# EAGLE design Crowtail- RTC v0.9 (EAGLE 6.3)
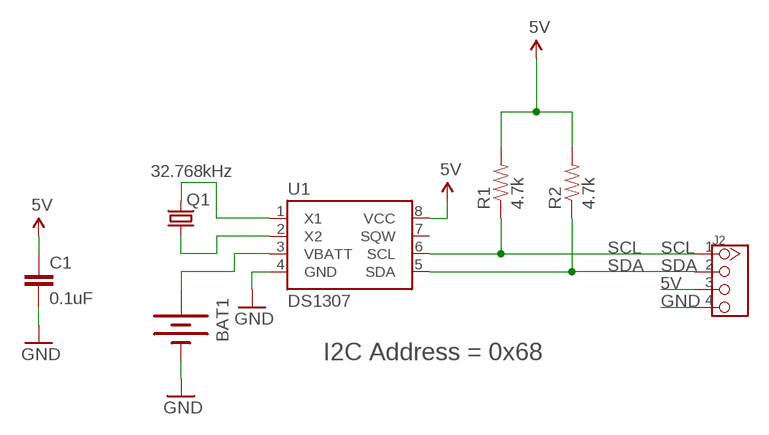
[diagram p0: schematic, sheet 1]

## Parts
BAT1  BATTERY12PTH  [BATTCON_12MM_PTH]
C1  0.1uF  0.1UF-25V(+80/-20%)(0603)  [0603-CAP]
J2  TWIG-4P-2.0-2.0  [4P-2.0]
Q1  32.768kHz  CRYSTAL32-SMD  [CRYSTAL-32KHZ-SMD]
R1  4.7k  4.7KOHM1/10W1%(0603)  [0603]
R2  4.7k  4.7KOHM1/10W1%(0603)  [0603]
U1  DS1307  DS1307SO8-TIGHT  [SO08-TIGHT]

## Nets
5V: C1.1 J2.3 R1.2 R2.2 U1.8(VCC)
GND: BAT1.GND(-) C1.2 J2.4 U1.4(GND)
N$1: Q1.X2 U1.1(X1)
N$2: Q1.X1 U1.2(X2)
N$4: BAT1.VCC@1(+) U1.3(VBATT)
SCL: J2.1 R1.1 U1.6(SCL)
SDA: J2.2 R2.1 U1.5(SDA)
Unconnected: U1.7(SQW)

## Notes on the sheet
- I2C Address = 0x68

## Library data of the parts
BAT1 = SparkFun-Electromechanical:BATTERY: Battery Holders
C1 = SparkFun-Capacitors:0.1UF-25V(+80/-20%)(0603): CAP-00810; PROD_ID: CAP-00810
J2 = Connector:TWIG-4P-2.0
Q1 = SparkFun-FreqCtrl:CRYSTAL: Various standard crystals. Proven footprints. Spark Fun Electronics SKU : COM-00534
R1 R2 = SparkFun-Resistors:4.7KOHM1/10W1%(0603): RES-07857; PROD_ID: RES-07857
U1 = SparkFun-FreqCtrl:DS1307: I2C real-time clock with battery backup.

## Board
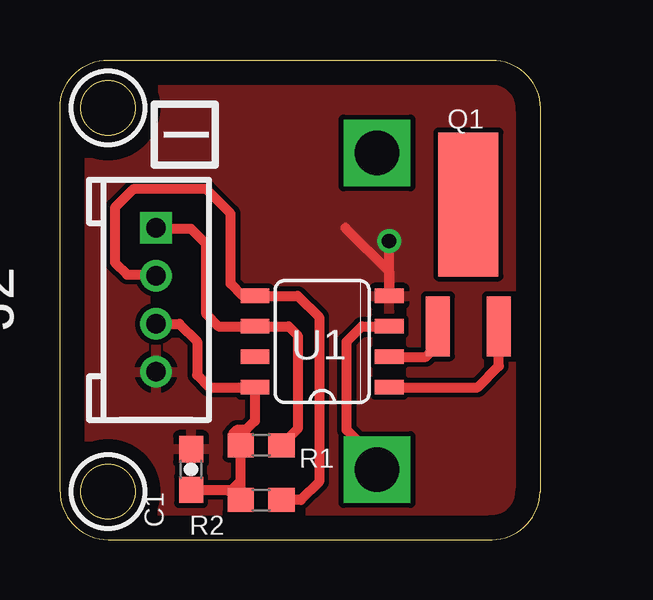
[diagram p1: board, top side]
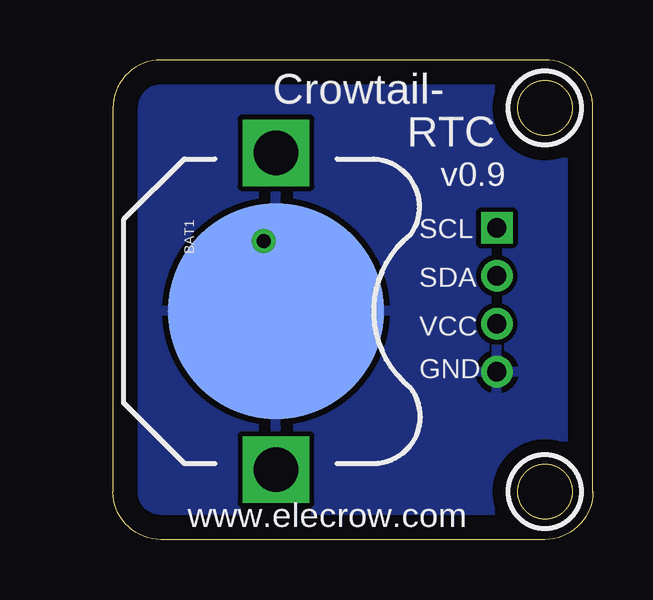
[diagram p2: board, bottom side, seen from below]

Size 20 x 20 mm. Coordinates in mm from the lower left corner, seen from the top.
Outline: 0,2 0,18 arc-90 2,20 18,20 arc-90 20,18 20,2 arc-90 18,0 2,0 arc-90 0,2
Outline: circle at 2,18 radius 1.14
Outline: circle at 2,2 radius 1.14
Copper layers (1*16): Top 0.035mm / dielectric 1.5mm / Bottom 0.035mm
Design rules "default *": minimum track width 10mil, minimum drill 24mil, track to track 8mil, track to pad 8mil, pad to pad 8mil, via to via 8mil, smd to smd 8mil, copper to edge 40mil, drill to drill 8mil, minimum pad ring 10mil, minimum via ring 8mil, stop-mask expansion 2mil, vias tented up to drill 100mil, thermal gap 10mil
tRestrict: area 0.5,16.5 to 3.5,19.5; area 0.5,0.5 to 3.5,3.5
bRestrict: area 0.5,16.5 to 3.5,19.5; area 0.5,0.5 to 3.5,3.5

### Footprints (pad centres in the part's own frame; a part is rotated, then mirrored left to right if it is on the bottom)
BATTCON_12MM_PTH = smd 9 x 9: GND 0,0 | drill 1.854 square: VCC@1 6.604,0; VCC@2 -6.604,0
0603-CAP = smd 1.1 x 1: 1 -0.85,0; 2 0.85,0
4P-2.0 = drill 0.8 pad 1.27 square: 1 -3,0 | drill 0.8 pad 1.27: 2 -1,0; 3 1,0; 4 3,0
CRYSTAL-32KHZ-SMD = smd 2.5 x 6: SHEILD 0,5.08 | smd 1 x 2.5: X1 -1.27,0; X2 1.27,0
0603 = smd 1.1 x 1: 1 -0.85,0; 2 0.85,0
SO08-TIGHT = smd 0.6 x 1.2: 1 -1.905,-2.8; 2 -0.635,-2.8; 3 0.635,-2.8; 4 1.905,-2.8; 5 1.905,2.8; 6 0.635,2.8; 7 -0.635,2.8; 8 -1.905,2.8

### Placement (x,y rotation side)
BAT1  13.21,9.53 270 bottom
C1  5.46,2.92 90 top
J2  4,10 270 top
Q1  17.02,8.89 0 top
R1  8.38,3.94 180 top
R2  8.38,1.65 180 top
U1  10.92,8.26 90 top

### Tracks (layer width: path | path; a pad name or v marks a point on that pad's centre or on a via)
5V
  Top 0.406: C1.1 7.11,2.07 R2.2 R1.2 7.62,4.03 7.62,4.45 7.75,4.57 | 7.75,4.57 8.12,4.95 U1.8 6.22,6.35 5.71,6.86 5.71,8.26 4.97,9 J2.3 | 7.75,4.57 7.37,4.57 7.24,4.45
GND  (via drill 0.6)
  Top 0.406: 11.89,13 13.72,11.18 U1.4 v13.72,12.44 v13.72,12.45
  Bottom 0.406: 14.48,12.57 14.35,12.45 v13.72,12.45 13.21,11.94 BAT1.GND
  pour Top: 0,20.32 20.32,20.32 20.32,0 0,0
  pour Top: 0,20.32 20.32,20.32 20.32,0 0,0
  pour Bottom: 20.32,20.32 20.32,0 0,0 0,20.32
N$1
  Top 0.406: U1.1 17.4,6.35 18.29,7.24 Q1.X2
N$2
  Top 0.406: U1.2 15.24,7.62 15.75,8.13 Q1.X1
N$3
  Top 0.406: 6.99,2.03 7.11,2.03 7.49,2.41
N$4
  Top 0.406: BAT1.VCC@1 13.21,3.3 11.94,4.57 11.94,8.26 12.57,8.89 U1.3
SCL
  Top 0.406: R1.1 9.91,4.61 9.91,8.51 9.53,8.89 U1.6 6.6,8.89 6.1,9.4 6.1,12.32 5.46,12.95 4.05,12.95 J2.1
SDA
  Top 0.406: R2.1 10.03,1.65 10.79,2.41 10.79,9.27 9.91,10.16 U1.5 7.62,10.16 7.11,10.67 7.11,13.59 6.1,14.61 3.05,14.61 2.29,13.84 2.29,11.56 2.79,11.05 3.95,11.05 J2.2

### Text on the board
tPlace: I
bPlace: Crowtail- | RTC | v0.9 | SCL | SDA | VCC | GND | www.elecrow.com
